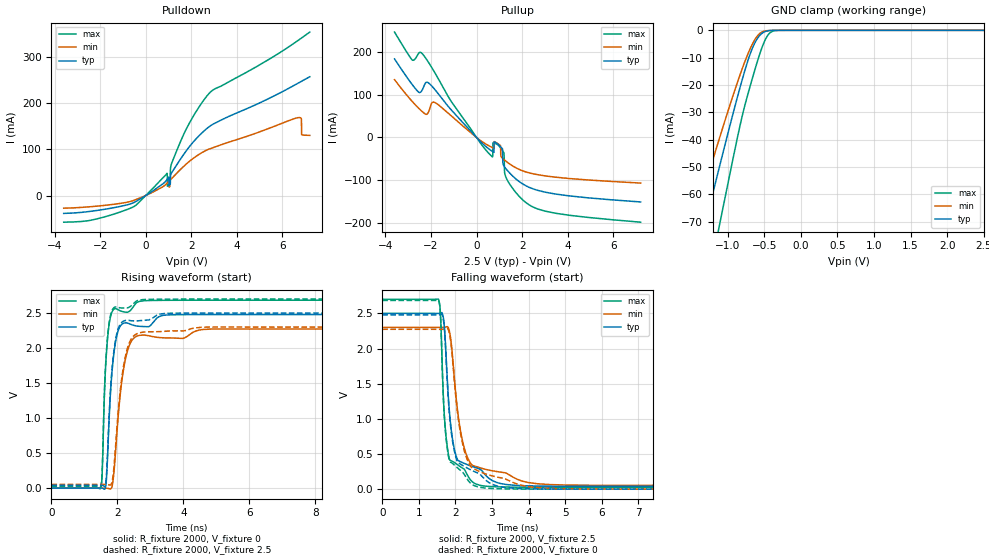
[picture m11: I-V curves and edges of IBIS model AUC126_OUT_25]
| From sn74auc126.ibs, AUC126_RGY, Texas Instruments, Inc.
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[Model]   AUC126_OUT_25
Model_type  3-state
Enable   Active-High
Vref =   0
Rref =   2000
Cref =   15p
Vmeas =   1.25
| variable   typ   min   max
C_comp   4.97pF   4.42pF   5.29pF
| C_pullup   6.30pF   0.06pF   11.35pF
| C_pulldown   6.37pF   5.04pF   15.83pF
| C_tri-state   4.97pF   4.42pF   5.29pF
[Temperature Range]   40   100   -40
| Ambient temperature   25   85   -40
[Voltage range]   2.5   2.3   2.7
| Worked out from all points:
|   slope of the pulldown table from 0 to 0.375 V, typ, clamps not added: 30.9 ohm
|   slope of the pullup table from 0 to 0.375 V, typ, clamps not added: 19.2 ohm
|   GND clamp passes 1 mA (typ) near -0.53 V on its own axis
|   rising waveform, R_fixture 2000, V_fixture 0: 20-80 % time 204ps typ, 299ps min, 144ps max; typ from 0 V to 2.48 V
|   falling waveform, R_fixture 2000, V_fixture 2.5: 20-80 % time 255ps typ, 365ps min, 172ps max; typ from 2.5 V to 0.04 V
|   rising waveform, R_fixture 2000, V_fixture 2.5: 20-80 % time 204ps typ, 299ps min, 143ps max; typ from 0.04 V to 2.5 V
|   falling waveform, R_fixture 2000, V_fixture 0: 20-80 % time 259ps typ, 372ps min, 173ps max; typ from 2.48 V to 0 V
[GND Clamp]
| AUC126_OUT_25
|   Voltage   I(typ)   I(min)   I(max)
-3.6V     -324.8mA   -272.6mA   -395.3mA
-1.515V   -93.62mA   -75.35mA   -124.4mA
-1.455V   -87.03mA   -69.89mA   -116.5mA
-1.295V   -69.56mA   -55.5mA    -95.38mA
-1.105V   -49.1mA    -38.82mA   -70.28mA
-850mV    -22.72mA   -17.71mA   -37.11mA
-725mV    -11.19mA   -8.712mA   -23.46mA
-625mV    -4.389mA   -3.231mA   -14.1mA
-525mV    -974.6uA   -541.7uA   -5.852mA
-435mV    -119.5uA   -65.92uA   -1.256mA
-325mV    -4.911uA   -4.228uA   -43.96uA
2.5V      725.8pA    175nA      1.045nA
[Pulldown]
| AUC126_OUT_25
|   Voltage   I(typ)   I(min)   I(max)
-3.6V     -38.75mA   -27.46mA   -57.79mA
-580mV    -16.57mA   -11.5mA    -25.48mA
935mV     34.57mA    26.63mA    48.15mA
950mV     35.58mA    27.35mA    20.2mA
1.075V    24.55mA    33.22mA    46.33mA
1.11V     47.04mA    35.44mA    65.44mA
1.62V     85.87mA    61.08mA    127.6mA
2.78V     149.1mA    100.7mA    221.4mA
6.695V    243.9mA    169mA      336.6mA
6.835V    247.7mA    165.4mA    341.5mA
6.84V     247.8mA    131.8mA    341.7mA
7.2V      257.6mA    130.5mA    354.4mA
[Pullup]
| AUC126_OUT_25
|   Voltage   I(typ)   I(min)   I(max)
-3.6V     183.2mA    134.8mA    245.7mA
-2.82V    123.1mA    83.81mA    180.7mA
-2.33V    117.1mA    57.9mA     192mA
-1.815V   110.7mA    81.11mA    149.5mA
510mV     -25.46mA   -18.52mA   -35.46mA
1.03V     -20.52mA   -18.17mA   -22.58mA
1.14V     -26.75mA   -48.47mA   -30.66mA
1.195V    -65.95mA   -51.04mA   -35.21mA
1.23V     -69.04mA   -52.63mA   -81.32mA
1.32V     -74.92mA   -56.52mA   -96.42mA
2.17V     -112.6mA   -80.39mA   -151.9mA
7.2V      -150.3mA   -106.2mA   -197.4mA
[Ramp]
| AUC126_OUT_25
| variable   typ   min   max
dV/dt_r   1.50/2.05E-10   1.37/3.01E-10   1.62/1.44E-10
dV/dt_f   1.48/2.56E-10   1.35/3.66E-10   1.61/1.73E-10
R_load = 2000
[Rising Waveform]
| AUC126_OUT_25
R_fixture =   2000
C_fixture =   0
L_fixture =   0
V_fixture =   0
V_fixture_min = 0
V_fixture_max = 0
|   Time   V(typ)   V(min)   V(max)
0s        11.11nV    33.4nV     1.97nV
1.505ns   578uV      55.92uV    10.05mV
1.54ns    -740.1uV   137.4uV    233.9mV
1.655ns   59.12mV    -329.9uV   1.841V
1.78ns    1.28V      -11.45mV   2.425V
1.865ns   1.807V     101.3mV    2.54V
1.96ns    2.13V      628.2mV    2.561V
2.22ns    2.359V     1.789V     2.515V
2.665ns   2.311V     2.182V     2.667V
20ns      2.479V     2.273V     2.683V
[Falling Waveform]
| AUC126_OUT_25
R_fixture =   2000
C_fixture =   0
L_fixture =   0
V_fixture =   2.5
V_fixture_min = 2.3
V_fixture_max = 2.7
|   Time   V(typ)   V(min)   V(max)
0s        2.5V       2.3V       2.7V
1.535ns   2.5V       2.3V       2.703V
1.595ns   2.503V     2.3V       2.451V
1.685ns   2.38V      2.3V       1.162V
1.825ns   1.178V     2.269V     452.8mV
1.98ns    551.7mV    1.527V     376.3mV
2.185ns   379.8mV    709.1mV    302.9mV
2.655ns   288.4mV    307.1mV    57.61mV
3.98ns    47.39mV    95.38mV    27.32mV
20ns      40.45mV    53.08mV    26.22mV
[Rising Waveform]
| AUC126_OUT_25
R_fixture =   2000
C_fixture =   0
L_fixture =   0
V_fixture =   2.5
V_fixture_min = 2.3
V_fixture_max = 2.7
|   Time   V(typ)   V(min)   V(max)
0s        40.42mV    53.07mV    26.21mV
1.505ns   40.99mV    53.13mV    36.64mV
1.54ns    39.69mV    53.21mV    265.3mV
1.605ns   26.37mV    53.58mV    1.352V
1.655ns   104.8mV    52.78mV    1.864V
1.78ns    1.321V     43.47mV    2.447V
1.955ns   2.148V     666.1mV    2.588V
2.21ns    2.39V      1.807V     2.572V
2.645ns   2.39V      2.215V     2.684V
20ns      2.5V       2.3V       2.7V
[Falling Waveform]
| AUC126_OUT_25
R_fixture =   2000
C_fixture =   0
L_fixture =   0
V_fixture =   0
V_fixture_min = 0
V_fixture_max = 0
|   Time   V(typ)   V(min)   V(max)
0s        2.479V     2.273V     2.683V
1.535ns   2.478V     2.273V     2.687V
1.595ns   2.481V     2.273V     2.432V
1.68ns    2.379V     2.273V     1.194V
1.82ns    1.181V     2.248V     442.2mV
1.975ns   534mV      1.517V     341.5mV
2.18ns    343.2mV    685.9mV    250.3mV
2.61ns    229.6mV    262.4mV    33.29mV
4.75ns    1.495mV    8.751mV    290.5uV
20ns      28.24uV    5.695uV    11.99uV
